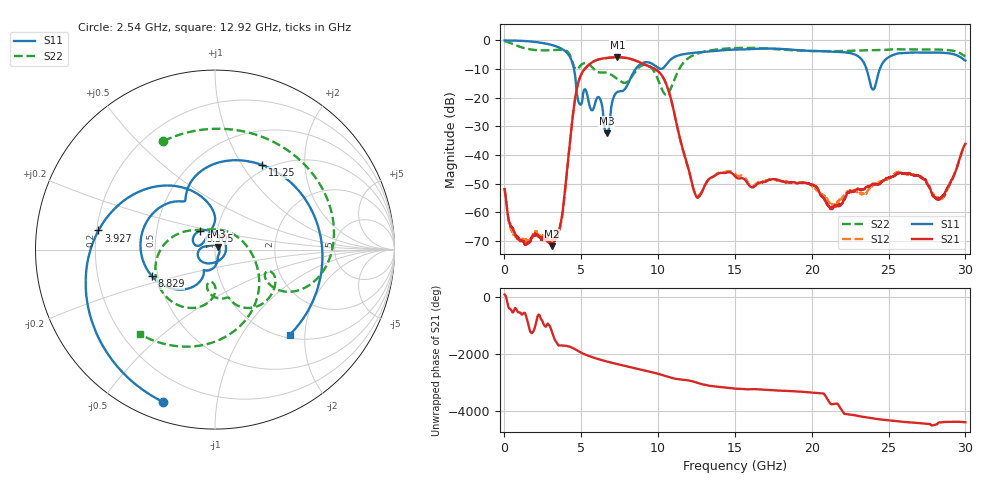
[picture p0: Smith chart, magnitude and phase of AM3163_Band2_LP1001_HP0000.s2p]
!Agilent Technologies,E8364B,MY43040894,A.07.50.67
!Agilent E8364B: A.07.50.67
!Date: Thursday, August 20, 2020 12:03:30
!Correction: S11(Full 2 Port(1,2))
!S21(Full 2 Port(1,2))
!S12(Full 2 Port(1,2))
!S22(Full 2 Port(1,2))
!S2P File: Measurements: S11, S21, S12, S22:
# Hz S  dB  R 50
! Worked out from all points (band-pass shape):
!   3201 points, 10 MHz to 30 GHz, reference 50 ohm
!   highest |S21| = -5.88 dB at 7.348 GHz (marker M1); lowest = -71.9 dB at 3.075 GHz (marker M2)
!   |S21| within 3 dB of the highest: 5.418 GHz to 9.35 GHz (3.932 GHz wide, 53.2 % of centre)
!   lowest |S11| = -32.5 dB at 6.655 GHz (marker M3), VSWR 1.05, Z = 51.7 + j1.68 ohm
!   |S11| at or under -10 dB: 4.527 GHz to 8.537 GHz (4.01 GHz wide, 61.4 % of centre); 23.57 GHz to 24.43 GHz (863.2 MHz wide, 3.6 % of centre)
!   |S22| runs from -19.0 to -0.2 dB; largest |S21 - S12| = 0.0041
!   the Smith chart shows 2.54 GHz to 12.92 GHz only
!   S11 on the Smith chart (normalised r, x): 2.54 GHz: 0.08, -0.71; 3.927 GHz: 0.21, +0.08; 5.305 GHz: 0.83, +0.18; 8.829 GHz: 0.46, -0.16; 11.25 GHz: 0.92, +1.23; 12.92 GHz: 1.07, -1.68
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1e7  -0.01 -3.0  -51.90 81.1  -51.75 -171.4  -0.21 -9.5
6.191719e8  -0.06 -25.5  -66.78 -123.4  -67.71 -169.3  -1.44 -78.7
1.322062e9  -0.21 -55.0  -71.04 155.1  -69.61 -22.7  -2.72 -149.3
2.540406e9  -0.95 -109.0  -69.54 134.0  -68.19 -21.5  -3.48 115.4
3.074603e9  -1.58 -135.6  -71.90 -120.6  -69.95 51.8  -3.39 77.6
3.927444e9  -3.64 170.7  -52.96 87.1  -53.71 88.3  -3.42 11.6
5.014581e9  -22.02 156.5  -11.66 -164.5  -11.66 -164.8  -8.45 -27.2
5.305109e9  -17.51 128.0  -9.48 125.1  -9.49 124.7  -7.88 -44.4
5.979884e9  -20.61 -127.5  -6.88 -3.1  -6.90 -3.2  -10.78 -73.0
6.654659e9  -32.46 43.0  -6.12 -106.4  -6.15 -106.5  -11.31 -86.4
7.348178e9  -18.01 -111.7  -5.88 160.4  -5.90 160.4  -13.48 -102.1
8.828934e9  -8.36 -157.6  -7.69 -25.6  -7.69 -25.9  -9.12 -111.6
1.000979e10  -9.64 125.3  -10.82 179.5  -10.83 179.3  -13.91 150.6
1.124688e10  -5.36 61.0  -30.19 -4.1  -30.36 -4.9  -11.35 -27.2
1.292444e10  -4.00 -48.6  -52.10 166.3  -51.93 167.3  -4.03 -131.4
1.5005e10  -3.18 -140.7  -47.45 21.4  -46.65 23.0  -2.66 150.2
1.776033e10  -2.90 95.9  -48.72 -46.3  -48.93 -47.7  -3.10 43.3
2.000958e10  -3.67 -19.1  -50.39 -117.9  -50.85 -117.8  -3.72 -40.5
2.398326e10  -17.19 -142.5  -50.14 56.9  -50.24 59.4  -3.40 -152.3
2.500479e10  -5.84 -135.9  -48.01 -10.8  -48.28 -9.9  -3.24 -177.0
2.84349e10  -4.27 104.0  -55.00 -83.4  -55.32 -77.9  -3.22 93.1
3e10  -7.02 44.1  -36.11 -79.5  -36.23 -81.1  -5.58 46.3
